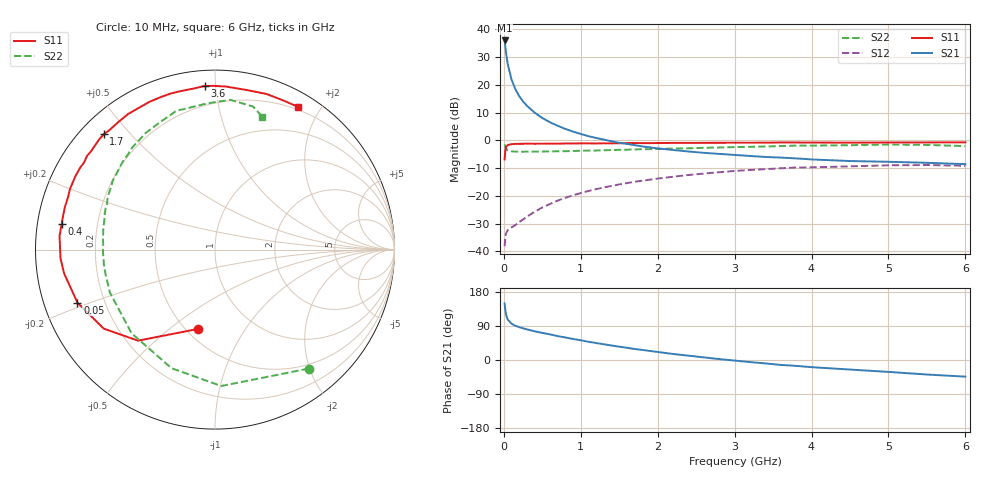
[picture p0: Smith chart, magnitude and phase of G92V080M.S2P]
! SIEMENS Small Signal Semiconductors
! BFG235
! Si NPN RF Bipolar Junction Transistor in SOT223
! VCE = 2 V  IC = 80 mA
! Common Emitter S-Parameters:  July  1994
# GHz  S  MA  R  50
!  f  S11  S21  S12  S22
! GHz  MAG  ANG  MAG  ANG  MAG  ANG  MAG  ANG
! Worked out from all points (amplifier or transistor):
!   40 points, 10 MHz to 6 GHz, reference 50 ohm
!   highest |S21| = 35.9 dB at 10 MHz (marker M1)
!   |S21| within 3 dB of that: start of sweep to 22.43 MHz
!   unconditionally stable (mu >= 1): 464.1 MHz to 1.557 GHz
!   at 200 MHz: K = 0.76, MSG = 22.7 dB, |S12| = -29.4 dB
!   at 1.5 GHz: K = 1.01, MAG = 6.8 dB, |S12| = -15.9 dB
!   at 6 GHz: K = 0.93, MSG = 0.3 dB, |S12| = -9.2 dB
!   S11 on the Smith chart (normalised r, x): 10 MHz: 0.57, -0.63; 50 MHz: 0.10, -0.18; 400 MHz: 0.07, +0.08; 1.7 GHz: 0.07, +0.42; 3.6 GHz: 0.08, +0.94; 6 GHz: 0.17, +1.72
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0.01  0.4523 -102.2  62.73 149.5  0.0124 61.4  0.8438 -51.8
0.02  0.6644 -130.2  47.39 130.1  0.0185 45.2  0.7607 -87.4
0.03  0.7602 -144.6  36.29 118.5  0.0212 37.6  0.7038 -110.2
0.05  0.8214 -158.9  23.73 106.9  0.0241 30.2  0.6581 -135.0
0.1  0.8514 -171.1  12.41 95.8  0.027 32.2  0.6328 -157.9
0.15  0.8621 -176.8  8.315 90.3  0.0298 37.9  0.625 -167.1
0.2  0.8631 -180.0  6.217 86.7  0.0337 42.8  0.6248 -172.1
0.25  0.8658 177.1  5.007 83.5  0.0375 47.1  0.6227 -175.6
0.3  0.8695 175.0  4.188 80.9  0.042 50.2  0.6243 -178.6
0.4  0.8661 170.6  3.15 75.8  0.0516 54.1  0.6237 177.4
0.5  0.8675 167.0  2.519 71.4  0.0617 55.9  0.6272 174.1
0.6  0.8693 164.0  2.107 67.6  0.0713 56.5  0.6306 171.1
0.7  0.8694 160.3  1.822 63.1  0.082 57.1  0.6345 168.4
0.9  0.8762 155.0  1.433 55.5  0.102 55.4  0.6413 163.7
1.1  0.879 148.6  1.184 48.0  0.1221 53.2  0.6521 159.0
1.7  0.8929 133.9  0.817 29.1  0.1791 43.6  0.6849 146.8
2.2  0.8973 122.7  0.668 15.9  0.2209 34.4  0.7101 136.5
3.2  0.9035 101.6  0.522 -5.5  0.2917 15.2  0.7619 117.4
3.6  0.9136 93.6  0.488 -13.0  0.3131 6.8  0.7866 109.1
4.5  0.9067 78.3  0.423 -25.2  0.3393 -9.1  0.8159 93.0
5.5  0.914 65.3  0.393 -38.3  0.358 -26.9  0.8249 75.1
6  0.9197 59.9  0.372 -43.9  0.3473 -33.5  0.7856 70.4
